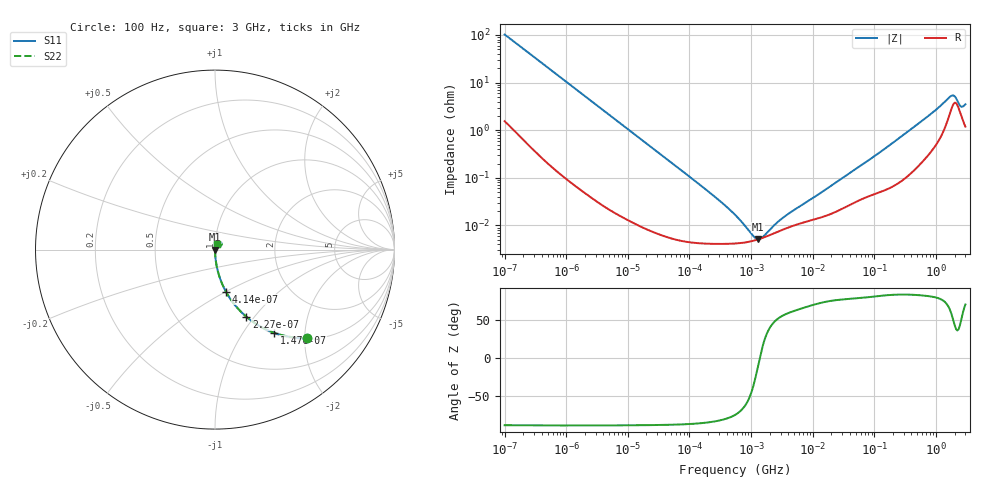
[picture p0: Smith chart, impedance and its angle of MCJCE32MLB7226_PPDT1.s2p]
! MCJCE32MLB7226_PPDT1  S-PARAMETER MODEL  ( Standard Model )
! Model Generated by TAIYO YUDEN Corporation (http://www.ty-top.com)
! Version 1.0
! TAIYO YUDEN Control No. 220601
! Copyright(c) 2015 TAIYO YUDEN CO.,LTD. All Rights Reserved.
! Product Description (link to TY-COMPAS)
! https://ds.yuden.co.jp/TYCOMPAS/or/detail?pn=MCJCE32MLB7226KPPDT1&u=M
! Products Name : Multilayer Ceramic Capacitors
! Characteristics :
!  Capacitance : 22 [uF] , Rated Voltage : 16 [V] , TCC : X7R
!  Case Size : 3.2 x 2.5 / 0.126 x 0.098 [mm/inch] , Thickness : 2.5 / 0.098 [mm/inch]
!  (Conditions: Temperature = 25 [degC] , DC Bias Voltage = 0 [V])
! External Node Assignments :
!  1  o---| |---o  2
! GND o---------o GND
! Frequency Range : 100Hz  -  3GHz  [ 401 STEP ]
# MHZ S RI R 50
! Freq[MHz].  S11 Real  S11 Imag  S21 Real  S21 Imag  S12 Real  S12 Imag  S22 Real  S22 Imag
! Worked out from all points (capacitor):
!   401 points, 100 Hz to 3 GHz, reference 50 ohm
!   read as one part in series: C = 15.5 uF near 109 Hz
!   lowest |Z| = 5.19 mohm at 1.295 MHz (marker M1)
!   series resonance near 1.387 MHz, so ESL is about 850 pH
!   S11 on the Smith chart (normalised r, x): 100 Hz: 1.03, -2.05; 147 Hz: 1.02, -1.40; 227 Hz: 1.01, -0.91; 414 Hz: 1.01, -0.50; 3 GHz: 1.02, +0.07
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0.0001  0.5119 -0.4924  0.4881 0.4924  0.4881 0.4924  0.5119 -0.4924
0.000147  0.33 -0.4635  0.67 0.4635  0.67 0.4635  0.33 -0.4635
0.000227  0.1748 -0.3739  0.8252 0.3739  0.8252 0.3739  0.1748 -0.3739
0.000414  0.061 -0.2344  0.939 0.2344  0.939 0.2344  0.061 -0.2344
0.000789  0.0182 -0.1291  0.9818 0.1291  0.9818 0.1291  0.0182 -0.1291
0.001788  0.00392 -0.0581  0.9961 0.0581  0.9961 0.0581  0.00392 -0.0581
0.005476  0.000566 -0.0192  0.9994 0.0192  0.9994 0.0192  0.000566 -0.0192
0.031977  7.62e-05 -0.00331  0.9999 0.00331  0.9999 0.00331  7.62e-05 -0.00331
0.231582  4.14e-05 -0.000447  1 0.000447  1 0.000447  4.14e-05 -0.000447
0.547723  4.19e-05 -0.000163  1 0.000163  1 0.000163  4.19e-05 -0.000163
0.740304  4.34e-05 -0.000101  1 0.000101  1 0.000101  4.34e-05 -0.000101
0.806856  4.41e-05 -8.57e-05  1 8.57e-05  1 8.57e-05  4.41e-05 -8.57e-05
1.295438  5.1e-05 -9.88e-06  0.9999 9.88e-06  0.9999 9.88e-06  5.1e-05 -9.88e-06
2.366551  6.88e-05 7.42e-05  0.9999 -7.42e-05  0.9999 -7.42e-05  6.88e-05 7.42e-05
4.141163  9.2e-05 0.000155  0.9999 -0.000155  0.9999 -0.000155  9.2e-05 0.000155
9.794414  0.00013 0.000345  0.9999 -0.000345  0.9999 -0.000345  0.00013 0.000345
175.1444  0.000628 0.00476  0.9994 -0.00476  0.9994 -0.00476  0.000628 0.00476
790.0314  0.00367 0.0206  0.9963 -0.0206  0.9963 -0.0206  0.00367 0.0206
1714.41  0.0256 0.0429  0.9744 -0.0429  0.9744 -0.0429  0.0256 0.0429
1950.712  0.0365 0.036  0.9635 -0.036  0.9635 -0.036  0.0365 0.036
2525.516  0.0214 0.0223  0.9786 -0.0223  0.9786 -0.0223  0.0214 0.0223
3000  0.0128 0.0323  0.9872 -0.0323  0.9872 -0.0323  0.0128 0.0323
